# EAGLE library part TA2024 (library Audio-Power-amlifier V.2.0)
The TA2 0 2 4 i s a 1 5 W / c h c o n t i n u o u s a v e r a g e t wo - c h a n n e l C l a s s - T D i g i t a l A u d i o Power A m p l i f i e r I C u s i n g T r i p a t h ’ s p r o p r i e t a r y D i g i t a l P o wer P r o c e s s i n g ™ t e c h n o l o g y. C l a s s - T a m p l i f i e r s o f f e r b o t h t h e a u d i o f i d e l i t y o f C l a s s - A B a n d t h e powe r e f f i c i e n c y o f C l a s s - D a m p l i f i e r s .
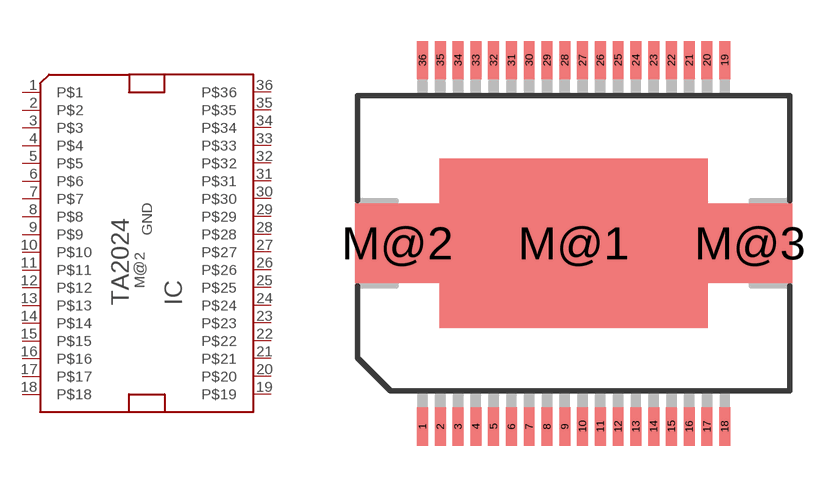
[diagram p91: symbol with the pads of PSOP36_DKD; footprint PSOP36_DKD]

Designator prefix IC

## TA2024  [PSOP36_DKD]
1  P$1
2  P$2
3  P$3
4  P$4
5  P$5
6  P$6
7  P$7
8  P$8
9  P$9
10  P$10
11  P$11
12  P$12
13  P$13
14  P$14
15  P$15
16  P$16
17  P$17
18  P$18
19  P$19
20  P$20
21  P$21
22  P$22
23  P$23
24  P$24
25  P$25
26  P$26
27  P$27
28  P$28
29  P$29
30  P$30
31  P$31
32  P$32
33  P$33
34  P$34
35  P$35
36  P$36
M@2  GND

## Footprint PSOP36_DKD (pad centres in mm)
36-Lead Power Small Ou t l i ne Package ( P S O P ) , s i m i l a r t o JEDEC out l i ne MO- 1 6 6 , var i a t i on AE:f
smd 0.4 x 1.4: 1 -5.525,-6.7; 2 -4.875,-6.7; 3 -4.225,-6.7; 4 -3.575,-6.7; 5 -2.925,-6.7; 6 -2.275,-6.7; 7 -1.625,-6.7; 8 -0.975,-6.7; 9 -0.325,-6.7; 10 0.325,-6.7; 11 0.975,-6.7; 12 1.625,-6.7; 13 2.275,-6.7; 14 2.925,-6.7; 15 3.575,-6.7; 16 4.225,-6.7; 17 4.875,-6.7; 18 5.525,-6.7; 19 5.525,6.7; 20 4.875,6.7; 21 4.225,6.7; 22 3.575,6.7; 23 2.925,6.7; 24 2.275,6.7; 25 1.625,6.7; 26 0.975,6.7; 27 0.325,6.7; 28 -0.325,6.7; 29 -0.975,6.7; 30 -1.625,6.7; 31 -2.275,6.7; 32 -2.925,6.7; 33 -3.575,6.7; 34 -4.225,6.7; 35 -4.875,6.7; 36 -5.525,6.7
smd 9.8 x 6.2: M@1 0,0
smd 3.1 x 2.9: M@2 -6.45,0; M@3 6.45,0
